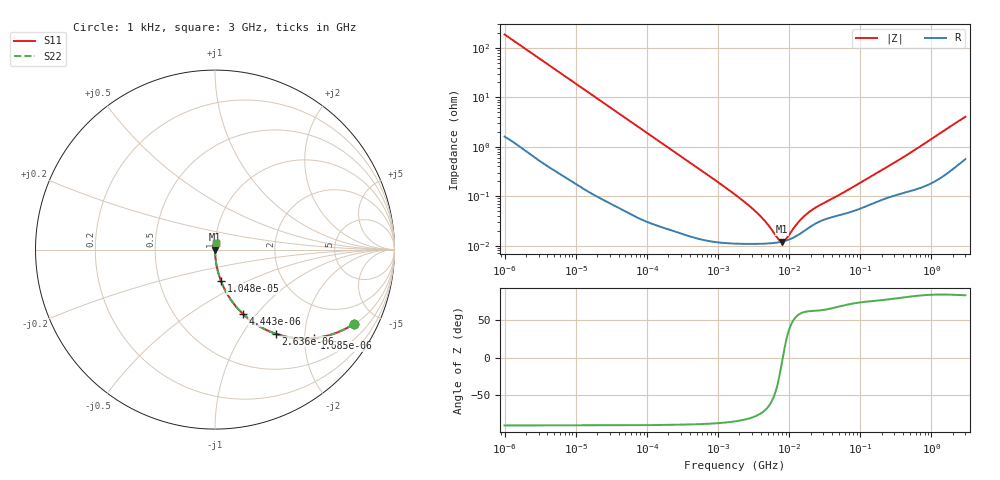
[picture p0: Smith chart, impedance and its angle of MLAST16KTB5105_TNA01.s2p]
! MLAST16KTB5105_TNA01  S-PARAMETER MODEL  ( Standard Model )
! Model Generated by TAIYO YUDEN Corporation (http://www.ty-top.com)
! Version 1.0
! TAIYO YUDEN Control No. 220601
! Copyright(c) 2009 TAIYO YUDEN CO.,LTD. All Rights Reserved.
! Product Description (link to TY-COMPAS)
! https://ds.yuden.co.jp/TYCOMPAS/or/detail?pn=MLAST16KTB5105KTNA01&u=M
! Products Name : Multilayer Ceramic Capacitors
! Characteristics :
!  Capacitance : 1 [uF] , Rated Voltage : 25 [V] , TCC : X5R
!  Case Size : 1.6 x 0.8 / 0.063 x 0.031 [mm/inch] , Thickness : 0.45 / 0.018 [mm/inch]
!  (Conditions: Temperature = 25 [degC] , DC Bias Voltage = 0 [V])
! External Node Assignments :
!  1  o---| |---o  2
! GND o---------o GND
! Frequency Range : 1kHz  -  3GHz  [ 401 STEP ]
# MHZ S RI R 50
! Freq[MHz].  S11 Real  S11 Imag  S21 Real  S21 Imag  S12 Real  S12 Imag  S22 Real  S22 Imag
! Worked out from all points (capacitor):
!   401 points, 1 kHz to 3 GHz, reference 50 ohm
!   read as one part in series: C = 852 nF near 1.077 kHz
!   lowest |Z| = 12.1 mohm at 7.989 MHz (marker M1)
!   series resonance near 8.144 MHz, so ESL is about 450 pH
!   S11 on the Smith chart (normalised r, x): 1 kHz: 1.03, -3.73; 1.685 kHz: 1.02, -2.22; 2.636 kHz: 1.01, -1.42; 4.443 kHz: 1.01, -0.85; 10.47 kHz: 1.00, -0.36; 3 GHz: 1.01, +0.08
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0.001  0.7745 -0.4136  0.2255 0.4136  0.2255 0.4136  0.7745 -0.4136
0.001205  0.7042 -0.452  0.2958 0.452  0.2958 0.452  0.7042 -0.452
0.001685  0.5515 -0.493  0.4485 0.493  0.4485 0.493  0.5515 -0.493
0.002636  0.3373 -0.4685  0.6627 0.4685  0.6627 0.4685  0.3373 -0.4685
0.004443  0.154 -0.3567  0.846 0.3567  0.846 0.3567  0.154 -0.3567
0.006451  0.0806 -0.2678  0.9194 0.2678  0.9194 0.2678  0.0806 -0.2678
0.010475  0.033 -0.1741  0.967 0.1741  0.967 0.1741  0.033 -0.1741
0.01216  0.025 -0.1514  0.975 0.1514  0.975 0.1514  0.025 -0.1514
0.033275  0.00391 -0.0569  0.9961 0.0569  0.9961 0.0569  0.00391 -0.0569
0.147855  0.000415 -0.013  0.9996 0.013  0.9996 0.013  0.000415 -0.013
1.732051  0.000111 -0.00108  0.9999 0.00108  0.9999 0.00108  0.000111 -0.00108
3.651041  0.000109 -0.000429  0.9999 0.000429  0.9999 0.000429  0.000109 -0.000429
4.919932  0.000111 -0.000253  0.9999 0.000253  0.9999 0.000253  0.000111 -0.000253
6.881678  0.000116 -8.19e-05  0.9999 8.19e-05  0.9999 8.19e-05  0.000116 -8.19e-05
7.414467  0.000118 -4.54e-05  0.9999 4.54e-05  0.9999 4.54e-05  0.000118 -4.54e-05
7.988506  0.000121 -9.25e-06  0.9999 9.25e-06  0.9999 9.25e-06  0.000121 -9.25e-06
8.606987  0.000124 2.69e-05  0.9999 -2.69e-05  0.9999 -2.69e-05  0.000124 2.69e-05
9.273352  0.000128 6.32e-05  0.9999 -6.32e-05  0.9999 -6.32e-05  0.000128 6.32e-05
14.50609  0.000178 0.000286  0.9998 -0.000286  0.9998 -0.000286  0.000178 0.000286
21.06097  0.000255 0.000466  0.9997 -0.000466  0.9997 -0.000466  0.000255 0.000466
256.0921  0.000971 0.00404  0.999 -0.00404  0.999 -0.00404  0.000971 0.00404
3000  0.00715 0.0395  0.9928 -0.0395  0.9928 -0.0395  0.00715 0.0395
